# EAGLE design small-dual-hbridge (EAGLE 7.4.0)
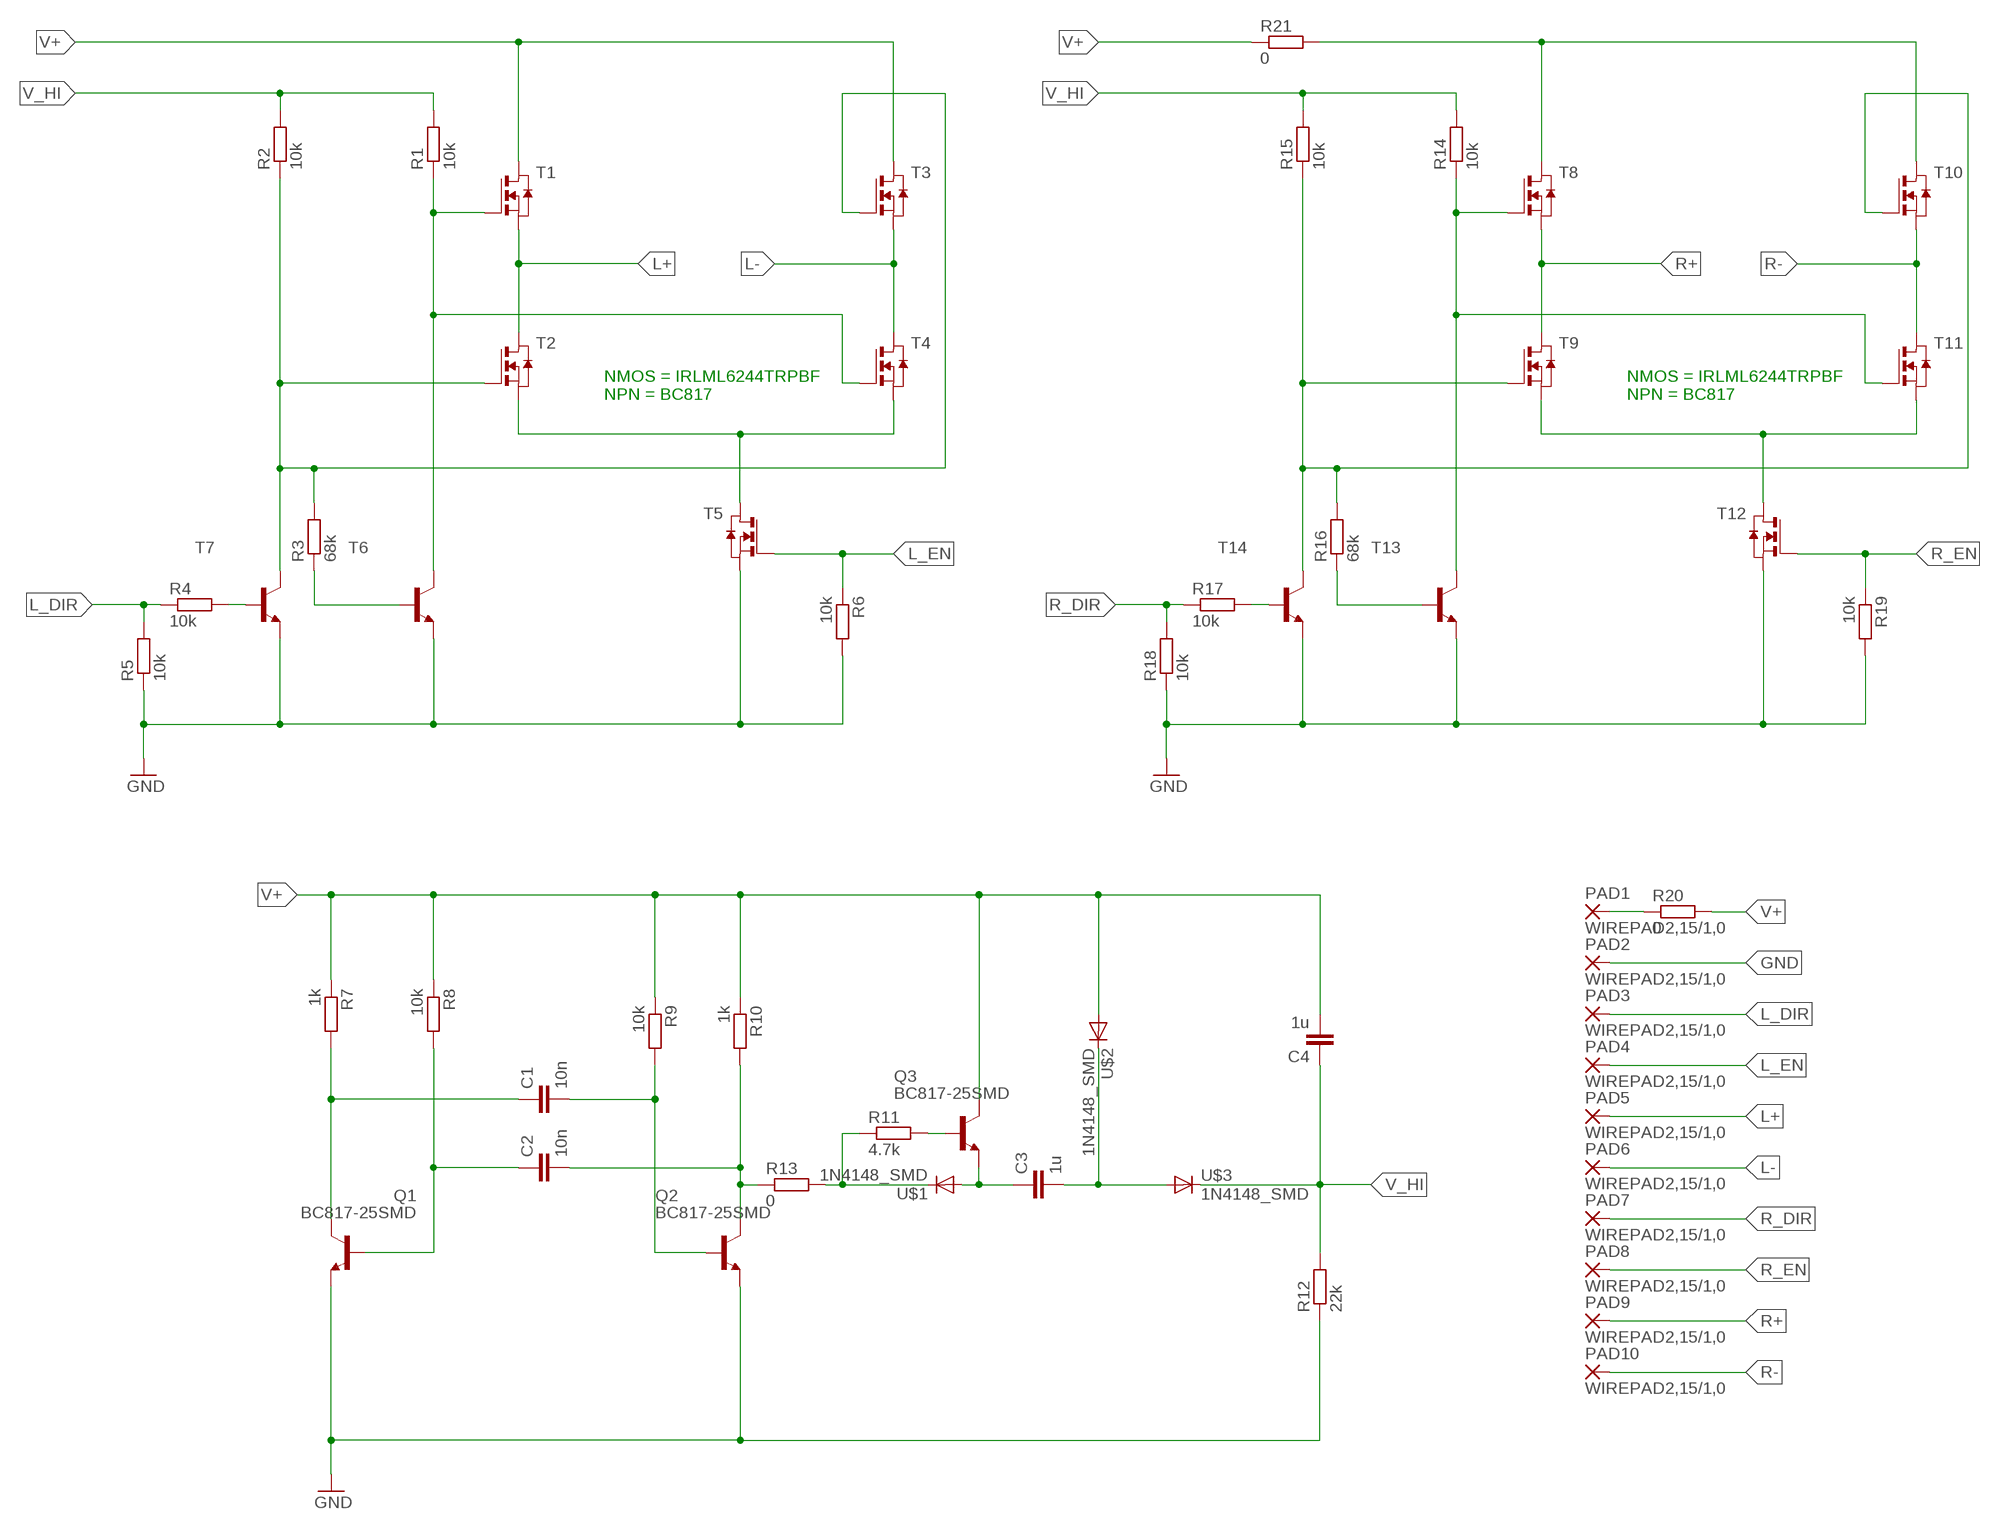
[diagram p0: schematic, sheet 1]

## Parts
C1  10n  C-EUC0805  [C0805]
C2  10n  C-EUC0805  [C0805]
C3  1u  C-EUC0805  [C0805]
C4  1u  C-EUC0805  [C0805]
PAD1  WIREPAD2,15/1,0  [2,15/1,0]
PAD2  WIREPAD2,15/1,0  [2,15/1,0]
PAD3  WIREPAD2,15/1,0  [2,15/1,0]
PAD4  WIREPAD2,15/1,0  [2,15/1,0]
PAD5  WIREPAD2,15/1,0  [2,15/1,0]
PAD6  WIREPAD2,15/1,0  [2,15/1,0]
PAD7  WIREPAD2,15/1,0  [2,15/1,0]
PAD8  WIREPAD2,15/1,0  [2,15/1,0]
PAD9  WIREPAD2,15/1,0  [2,15/1,0]
PAD10  WIREPAD2,15/1,0  [2,15/1,0]
Q1  BC817-25SMD  [SOT23-BEC]
Q2  BC817-25SMD  [SOT23-BEC]
Q3  BC817-25SMD  [SOT23-BEC]
R1  10k  R-EU_R0805  [R0805]
R2  10k  R-EU_R0805  [R0805]
R3  68k  R-EU_R0805  [R0805]
R4  10k  R-EU_R0805  [R0805]
R5  10k  R-EU_R0805  [R0805]
R6  10k  R-EU_R0805  [R0805]
R7  1k  R-EU_R0805  [R0805]
R8  10k  R-EU_R0805  [R0805]
R9  10k  R-EU_R0805  [R0805]
R10  1k  R-EU_R0805  [R0805]
R11  4.7k  R-EU_R0805  [R0805]
R12  22k  R-EU_R0805  [R0805]
R13  0  R-EU_R1206  [R1206]
R14  10k  R-EU_R0805  [R0805]
R15  10k  R-EU_R0805  [R0805]
R16  68k  R-EU_R0805  [R0805]
R17  10k  R-EU_R0805  [R0805]
R18  10k  R-EU_R0805  [R0805]
R19  10k  R-EU_R0805  [R0805]
R20  0  R-EU_R1206  [R1206]
R21  0  R-EU_R1206  [R1206]
T1  NMOSSOT23  [SOT-23]
T2  NMOSSOT23  [SOT-23]
T3  NMOSSOT23  [SOT-23]
T4  NMOSSOT23  [SOT-23]
T5  NMOSSOT23  [SOT-23]
T6  BC817-25-NPN-SOT23-BEC  [SOT23-BEC]
T7  BC817-25-NPN-SOT23-BEC  [SOT23-BEC]
T8  NMOSSOT23  [SOT-23]
T9  NMOSSOT23  [SOT-23]
T10  NMOSSOT23  [SOT-23]
T11  NMOSSOT23  [SOT-23]
T12  NMOSSOT23  [SOT-23]
T13  BC817-25-NPN-SOT23-BEC  [SOT23-BEC]
T14  BC817-25-NPN-SOT23-BEC  [SOT23-BEC]
U$1  1N4148_SMD  [1206]
U$2  1N4148_SMD  [1206]
U$3  1N4148_SMD  [1206]

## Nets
GND: PAD2.1(P) Q1.E Q2.E R5.1 R6.2 R12.1 R18.1 R19.2 T5.2(S) T6.E T7.E T12.2(S) T13.E T14.E
L+: PAD5.1(P) T1.2(S) T2.1(D)
L-: PAD6.1(P) T3.2(S) T4.1(D)
L_DIR: PAD3.1(P) R4.1 R5.2
L_EN: PAD4.1(P) R6.1 T5.3(G)
N$1: PAD1.1(P) R20.1
N$2: R21.2 T8.1(D) T10.1(D)
N$3: T2.2(S) T4.2(S) T5.1(D)
N$5: R1.1 T1.3(G) T4.3(G) T6.C
N$6: C1.1 Q1.C R7.2
N$7: R2.1 R3.2 T2.3(G) T3.3(G) T7.C
N$9: C2.2 Q2.C R10.2 R13.1
N$10: R3.1 T6.B
N$11: R4.2 T7.B
N$12: C1.2 Q2.B R9.2
N$13: C2.1 Q1.B R8.2
N$14: Q3.B R11.2
N$15: C3.1 Q3.E U$1.1(A)
N$16: C3.2 U$2.2(C) U$3.1(A)
N$17: T9.2(S) T11.2(S) T12.1(D)
N$18: R11.1 R13.2 U$1.2(C)
N$19: R14.1 T8.3(G) T11.3(G) T13.C
N$20: R15.1 R16.2 T9.3(G) T10.3(G) T14.C
N$21: R16.1 T13.B
N$22: R17.2 T14.B
R+: PAD9.1(P) T8.2(S) T9.1(D)
R-: PAD10.1(P) T10.2(S) T11.1(D)
R_DIR: PAD7.1(P) R17.1 R18.2
R_EN: PAD8.1(P) R19.1 T12.3(G)
V+: C4.2 Q3.C R7.1 R8.1 R9.1 R10.1 R20.2 R21.1 T1.1(D) T3.1(D) U$2.1(A)
V_HI: C4.1 R1.2 R2.2 R12.2 R14.2 R15.2 U$3.2(C)

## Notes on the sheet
- NMOS = IRLML6244TRPBF
  NPN = BC817
- NMOS = IRLML6244TRPBF
  NPN = BC817

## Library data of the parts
C1-C4 = rcl:C-EU: CAPACITOR, European symbol
PAD1-PAD10 = wirepad:WIREPAD: Wire PAD connect wire on PCB
Q1-Q3 = transistor-npn:BC817*: NPN Transistor
R1-R21 = rcl:R-EU_: RESISTOR, European symbol
T1-T5 T8-T12 = zetex:NMOSSOT23: MOS FET; OC_FARNELL: unknown; OC_NEWARK: unknown
T6 T7 T13 T14 = transistor:*-NPN-: NPN Transistror BF959 corrected 2008.03.06
U$1-U$3 = mylib:1N4148_SMD

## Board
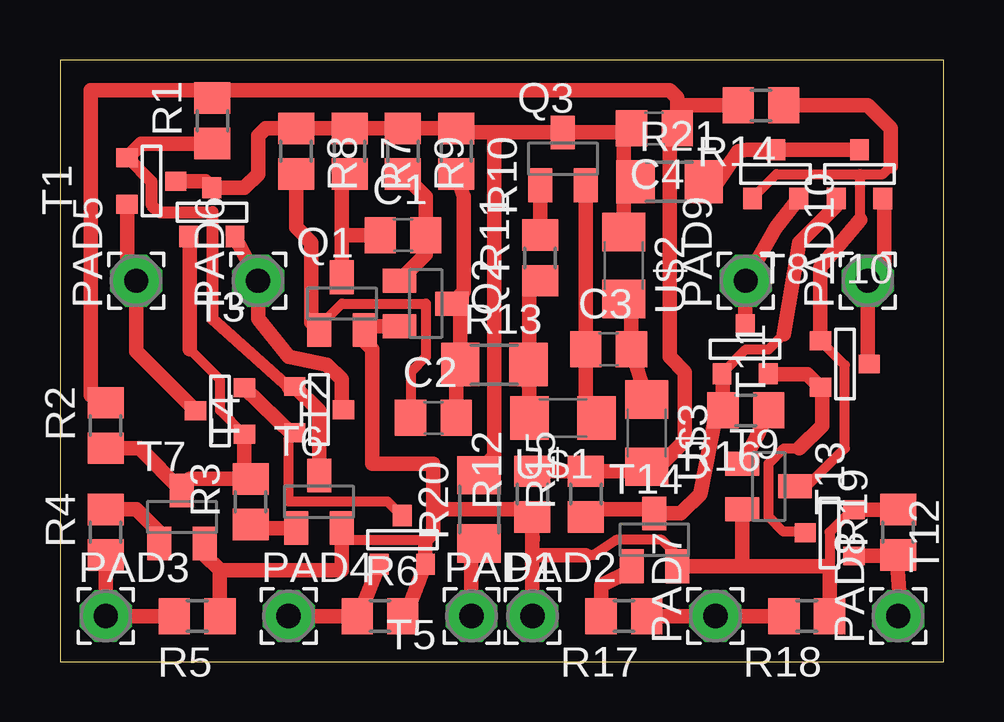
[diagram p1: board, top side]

Size 36.82 x 25.07 mm. Coordinates in mm from the lower left corner, seen from the top.
Outline: 0,0 36.82,0 36.82,25.07 0,25.07 0,0
Copper layers (1*16): Top 0.035mm / dielectric 1.5mm / Bottom 0.035mm
Design rules "default": minimum track width 10mil, minimum drill 24mil, track to track 8mil, track to pad 8mil, pad to pad 8mil, via to via 8mil, smd to smd 8mil, copper to edge 40mil, drill to drill 8mil, minimum pad ring 10mil, minimum via ring 8mil, stop-mask expansion 4mil, vias tented up to drill 0mil, thermal gap 10mil

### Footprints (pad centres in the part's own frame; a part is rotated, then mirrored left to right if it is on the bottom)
C0805 = smd 1.3 x 1.5: 1 -0.95,0; 2 0.95,0
2,15/1,0 = drill 1.016 pad 2.159 octagon: 1 0,0
SOT23-BEC = smd 1 x 1.4: B -0.95,-1.1; C 0,1.1; E 0.95,-1.1
R0805 = smd 1.3 x 1.5: 1 -0.95,0; 2 0.95,0
R1206 = smd 1.6 x 1.803: 1 -1.422,0; 2 1.422,0
SOT-23 = smd 0.787 x 0.889: 1 0.025,-1.016; 2 -0.94,1.016; 3 0.991,1.016
1206 = smd 1.6 x 1.8: 1 -1.4,0; 2 1.4,0

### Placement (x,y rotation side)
C1  14.29,17.78 0 top
C2  15.56,10.16 0 top
C3  22.86,13.02 0 top
C4  24.77,22.23 180 top
PAD1  17.14,1.91 0 top
PAD2  19.68,1.91 0 top
PAD3  1.91,1.91 0 top
PAD4  9.53,1.91 0 top
PAD5  3.17,15.88 90 top
PAD6  8.26,15.88 90 top
PAD7  27.3,1.91 90 top
PAD8  34.92,1.91 90 top
PAD9  28.57,15.88 90 top
PAD10  33.66,15.88 90 top
Q1  11.75,14.92 0 top
Q2  15.24,14.92 270 top
Q3  20.95,20.95 0 top
R1  6.35,22.54 90 top
R2  1.91,9.84 90 top
R3  7.94,6.67 90 top
R4  1.91,5.4 90 top
R5  5.71,1.91 180 top
R6  13.34,1.91 0 top
R7  12.06,21.27 270 top
R8  9.84,21.27 270 top
R9  14.29,21.27 270 top
R10  16.51,21.27 270 top
R11  20,16.83 90 top
R12  19.68,6.99 90 top
R13  18.1,12.38 0 top
R14  29.21,23.18 180 top
R15  21.91,6.99 90 top
R16  28.57,10.48 180 top
R17  23.5,1.91 180 top
R18  31.11,1.91 180 top
R19  34.92,5.4 90 top
R20  17.46,6.35 90 top
R21  25.4,20 0 top
T1  3.81,20 90 top
T2  6.67,10.48 270 top
T3  6.35,18.73 180 top
T4  10.79,10.48 90 top
T5  14.29,5.08 180 top
T6  10.79,6.67 0 top
T7  5.08,6.03 0 top
T8  29.84,20.32 180 top
T9  28.57,13.02 180 top
T10  33.34,20.32 180 top
T11  32.7,12.38 90 top
T12  32.07,5.4 270 top
T13  29.53,7.3 270 top
T14  24.77,5.08 0 top
U$1  20.95,10.16 180 top
U$2  23.5,16.51 270 top
U$3  24.45,9.53 270 top

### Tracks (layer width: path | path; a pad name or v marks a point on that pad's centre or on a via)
GND
  Top 0.406: 11.74,5.08 15.21,5.08 15.23,5.07 | T14.E 25.71,4.45 25.08,5.08 23.18,5.08 22.23,4.45 21.91,4.45 | 33.01,6.34 32.07,5.4 32.07,3.49
  Top 0.61: R6.2 14.28,1.6 T5.2 15.23,5.07 15.56,5.4 15.56,6.35 | 25.57,4.13 T14.E 28.57,3.98 | R19.2 34.91,6.34 T12.2 33.01,6.34 | 12.87,13.97 Q1.E | 19.68,5.72 R12.1 19.68,5.4 19.69,5.08 | 19.68,5.72 19.05,6.35 15.56,6.35 | 15.56,6.35 15.56,8.26 13.02,8.26 13.02,13.02 12.7,13.34 Q1.E | T6.E 11.74,5.08 11.74,3.81 9.53,3.81 6.67,3.81 | R5.1 6.67,3.81 | PAD2.1 19.68,3.81 19.68,4.76 | 19.68,4.76 19.68,5.72 | R18.1 32.06,3.18 32.07,3.18 32.07,3.49 32.07,3.81 31.9,3.98 28.57,3.98 | 21.91,4.45 19.68,4.45 19.68,4.76 | T13.E 28.43,4.13 28.57,3.98 | T7.E 6.03,4.45 6.67,3.81 | Q2.E 12.85,13.97 Q1.E
L+
  Top 0.61: T2.1 3.17,12.93 PAD5.1 2.79,16.26 T1.2
L-
  Top 0.61: T4.1 11.73,10.58 11.73,11.76 11.11,12.38 9.53,12.7 8.26,14.29 PAD6.1 8.24,15.89 T3.2
L_DIR
  Top 0.61: R4.1 PAD3.1 R5.2
L_EN
  Top 0.61: T5.3 12.34,1.63 R6.1 PAD4.1
N$1
  Top 0.61: PAD1.1 17.14,4.61 R20.1
N$2
  Top 0.61: T10.1 T8.1 28.64,21.34 28.26,21.27 27.3,19.85 R21.2
N$3
  Top 0.406: 14.22,6.1 13.65,6.67 9.53,6.67 9.53,9.28 9.7,9.46 T4.2
  Top 0.508: T4.2 9.78,9.46
  Top 0.61: T5.1 14.22,6.1 14.29,6.03 | 9.75,9.51 T4.2 | T2.2 9.7,9.46
N$5
  Top 0.508: T1.3 2.82,20.99 3.81,20 3.81,19.05 4.13,18.73 6.35,18.73 6.35,14.29 9.53,11.43
  Top 0.61: 9.53,11.43 9.74,11.43 T4.3 10.79,10.45 T6.C | R1.1 3.39,21.59 T1.3
N$6
  Top 0.61: Q1.C 11.75,17.78 | 11.75,17.78 11.75,20 R7.2 | C1.1 11.75,17.78
N$7
  Top 0.406: T2.3 7.66,9.49 6.67,10.48 6.67,11.75 5.4,13.02
  Top 0.61: T3.3 5.4,17.44 5.4,13.02 | T2.3 7.68,7.87 R3.2 6.03,7.62 5.4,7.62 5.25,7.45 T7.C 3.32,8.89 R2.1
N$9
  Top 0.61: 16.51,15.07 Q2.C | C2.2 16.51,11.58 R13.1 16.68,14.59 Q2.C | R10.2 16.83,19.37 16.83,15.41 Q2.C
N$10
  Top 0.61: T6.B 7.79,5.57 R3.1
N$11
  Top 0.61: R4.2 3.18,6.35 4.13,5.4 T7.B
N$12
  Top 0.61: 13.97,15.72 Q2.B | 14.29,16.05 Q2.B | R9.2 15.24,19.37 C1.2 15.24,16.97 Q2.B
N$13
  Top 0.406: Q1.B 10.8,13.97 11.75,14.92 15.24,14.92 15.24,12.7 14.61,12.06 C2.1
  Top 0.61: 10.63,13.97 Q1.B 10.48,14.14 10.48,17.46 9.84,18.1 R8.2 | C2.1
N$14
  Top 0.61: Q3.B R11.2
N$15
  Top 0.61: Q3.E 21.91,10.79 | 21.91,10.79 21.91,10.61 U$1.1 | C3.1 21.91,10.8 21.91,10.79
N$16
  Top 0.61: U$2.2 23.81,14.79 C3.2 U$3.1
N$17
  Top 0.406: 31.09,5.42 30.14,5.42 29.53,6.03 29.53,8.26 30.16,8.89 30.8,8.89
  Top 0.61: T12.1 31.09,5.42 | T9.2 29.53,11.99 31.14,11.99 T11.2 31.75,11.38 31.75,9.84 30.8,8.89
N$18
  Top 0.61: 19.55,11.08 19.55,15.43 R11.1 | U$1.2 19.55,11.08 | 19.55,11.08 R13.2
N$19
  Top 0.406: T13.C 31.11,7.3 32.7,8.89 32.7,12.36 T11.3 | 28.85,19.33 29.84,20.32 33.34,20.32 | 33.34,20.32 34.29,20.32 34.61,20.64 | 33.34,18.41 33.34,20.32
  Top 0.61: T8.3 28.85,19.33 | T11.3 31.69,16.45 33.34,18.41 | R14.1 33.66,23.18 34.61,22.23 34.61,20.64
N$20
  Top 0.406: T9.3 27.58,12.03 28.57,13.02 29.53,13.02 30.16,13.65
  Top 0.61: T10.3 32.32,18.99 30.8,17.46 30.16,13.65 | T9.3 27.58,12.11 R16.2 27.62,10.79 27.3,10.16 26.67,6.99 25.86,6.18 T14.C 24.59,6.35 22.54,6.35 22.23,6.04 R15.1
N$21
  Top 0.61: T13.B 29.04,9.38 R16.1
N$22
  Top 0.61: R17.2 22.55,3.18 23.81,3.81 23.96,4.13 T14.B
R+
  Top 0.61: T9.1 28.55,15.85 PAD9.1 29.83,18.09 T8.2
R-
  Top 0.61: T10.2 34.35,19.23 34.35,16.57 PAD10.1 33.66,12.47 T11.1
R_DIR
  Top 0.61: R17.1 PAD7.1 R18.2
R_EN
  Top 0.61: PAD8.1 34.92,2.54 34.97,2.9 34.88,4.09 R19.1 34.88,4.41 T12.3
V+
  Top 0.61: 18.41,22.05 Q3.C 23.64,22.05 C4.2 23.5,21.91 23.5,19.37 | 18.41,22.05 16.02,22.05 R10.1 R9.1 R7.1 R8.1 8.57,22.23 8.26,21.91 8.26,20.32 7.68,19.75 T3.1 6.04,20.03 T1.1 | 23.5,19.37 U$2.1 | R20.2 17.14,7.62 18.1,8.57 18.1,21.74 18.41,22.05 | R21.1 23.5,19.37
V_HI
  Top 0.61: C4.1 25.71,23.18 | 25.71,23.18 25.71,23.5 25.4,23.81 6.99,23.81 | 6.99,23.81 1.27,23.81 1.27,11.11 R2.2 | C4.1 25.71,21.91 | R1.2 6.35,23.81 6.99,23.81 | R14.2 25.71,23.18 | R12.2 R15.2 23.81,7.93 24.45,7.94 24.58,8.38 U$3.2 24.95,8.12 26.04,9.21 26.04,12.06 25.4,12.7 25.4,21.91 C4.1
